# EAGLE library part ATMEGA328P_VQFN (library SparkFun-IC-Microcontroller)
Atmel 328P QFN part not in catalog
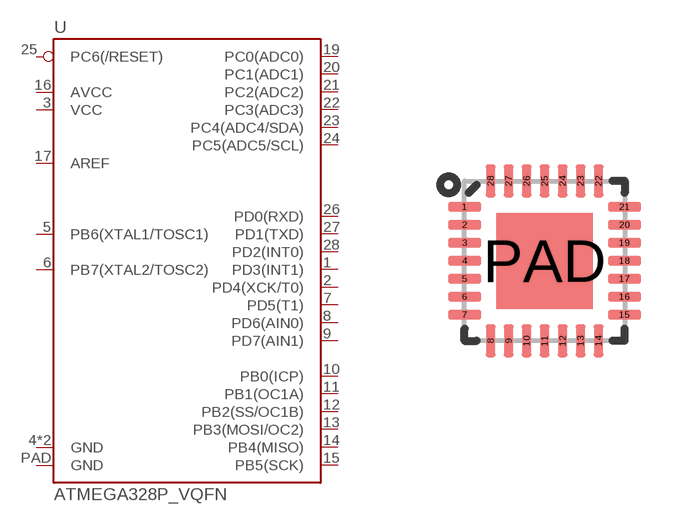
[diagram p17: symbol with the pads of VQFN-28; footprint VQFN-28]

Designator prefix U

## ATMEGA328P_VQFNVQFN  [VQFN-28]
1  PD3(INT1)
2  PD4(XCK/T0)
3  VCC
4  GND
5  PB6(XTAL1/TOSC1)
6  PB7(XTAL2/TOSC2)
7  PD5(T1)
8  PD6(AIN0)
9  PD7(AIN1)
10  PB0(ICP)
11  PB1(OC1A)
12  PB2(SS/OC1B)
13  PB3(MOSI/OC2)
14  PB4(MISO)
15  PB5(SCK)
16  AVCC
17  AREF
18  GND
19  PC0(ADC0)
20  PC1(ADC1)
21  PC2(ADC2)
22  PC3(ADC3)
23  PC4(ADC4/SDA)
24  PC5(ADC5/SCL)
25  PC6(/RESET)
26  PD0(RXD)
27  PD1(TXD)
28  PD2(INT0)
PAD  GND

## Footprint VQFN-28 (pad centres in mm)
smd 0.82 x 0.24: 1 -2,1.35; 2 -2,0.9; 3 -2,0.45; 4 -2,0; 5 -2,-0.45; 6 -2,-0.9; 7 -2,-1.35; 15 2,-1.35; 16 2,-0.9; 17 2,-0.45; 18 2,0; 19 2,0.45; 20 2,0.9; 21 2,1.35
smd 0.24 x 0.82: 8 -1.35,-2; 9 -0.9,-2; 10 -0.45,-2; 11 0,-2; 12 0.45,-2; 13 0.9,-2; 14 1.35,-2; 22 1.35,2; 23 0.9,2; 24 0.45,2; 25 0,2; 26 -0.45,2; 27 -0.9,2; 28 -1.35,2
smd 2.4 x 2.4: PAD 0,0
